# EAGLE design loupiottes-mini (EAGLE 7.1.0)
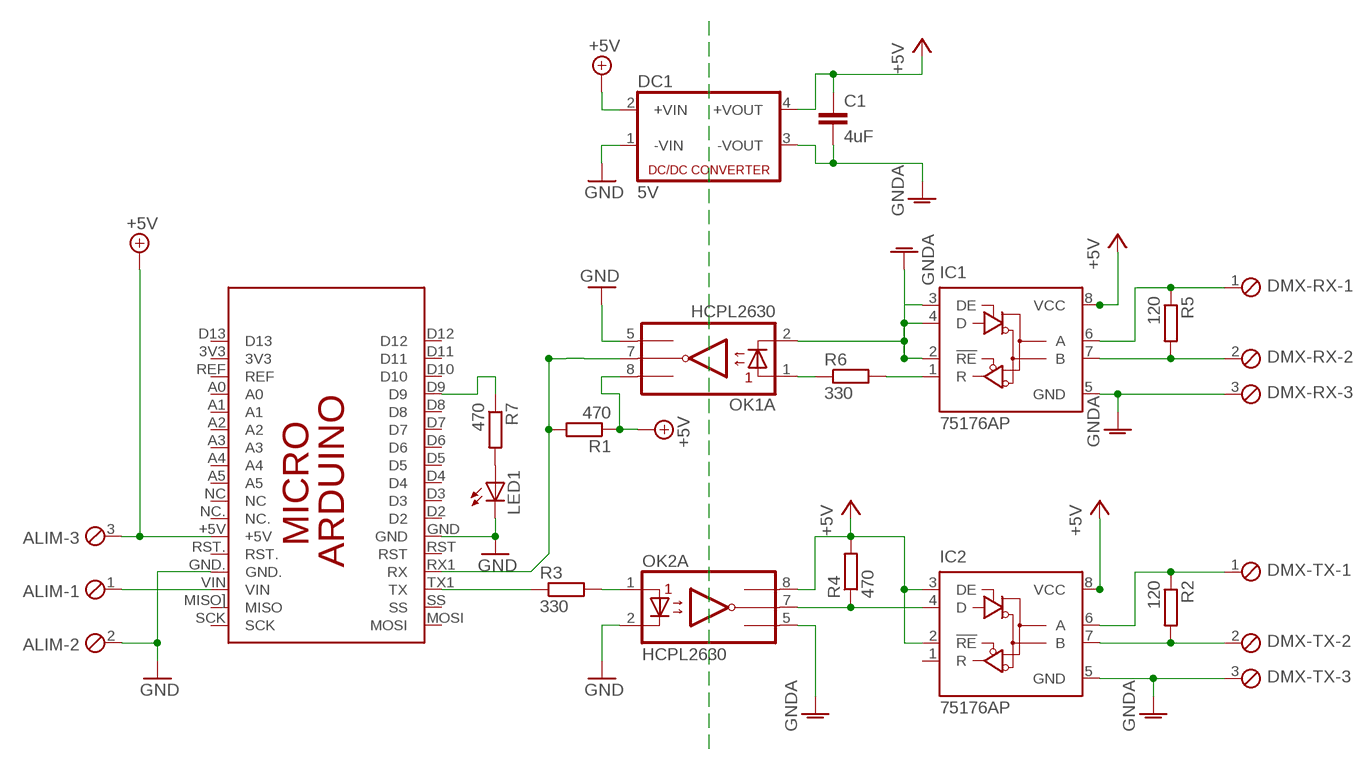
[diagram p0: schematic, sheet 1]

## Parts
ALIM  MPT3  [3POL254]
C1  4uF  C-EU025-024X044  [C025-024X044]
DC1  5V  NME  [NME]
DMX-RX  MPT3  [3POL254]
DMX-TX  MPT3  [3POL254]
IC1  75176AP  [DIL08]
IC2  75176AP  [DIL08]
LED1  LED3MM  [LED3MM]
OK1  HCPL2630  [DIL08]
OK2  HCPL2630  [DIL08]
PCB1  ARDUINO_MICRO  [ARDUINO_MICRO]
R1  470  R-EU_0207/10  [0207/10]
R2  120  R-EU_0207/10  [0207/10]
R3  330  R-EU_0207/10  [0207/10]
R4  470  R-EU_0207/10  [0207/10]
R5  120  R-EU_0207/10  [0207/10]
R6  330  R-EU_0207/10  [0207/10]
R7  470  R-EU_0207/10  [0207/10]

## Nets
+5V: ALIM.3 DC1.2(+VIN) OK1.8(A:VCC) PCB1.+5V R1.1
+5V-ISO: C1.1 DC1.4(+VOUT) IC1.8(VCC) IC2.2(!RE) IC2.3(DE) IC2.8(VCC) OK2.8(A:VCC) R4.2 ; supply symbol labelled +5V
GND: ALIM.2 DC1.1(-VIN) LED1.K(C) OK1.5(A:GND) OK2.2(A:C1) PCB1.GND PCB1.GND.
GND-ISO: C1.2 DC1.3(-VOUT) DMX-RX.3 DMX-TX.3 IC1.2(!RE) IC1.3(DE) IC1.4(D) IC1.5(GND) IC2.5(GND) OK1.2(A:C1) OK2.5(A:GND) ; supply symbol labelled GNDA
N$1: PCB1.TX1(TX) R3.1
N$2: OK2.1(A:A1) R3.2
N$3: OK1.7(A:VO1) PCB1.RX1(RX) R1.2
N$4: IC2.4(D) OK2.7(A:VO1) R4.1
N$5: DMX-TX.1 IC2.6(A) R2.1
N$6: DMX-TX.2 IC2.7(B) R2.2
N$7: DMX-RX.1 IC1.6(A) R5.1
N$8: DMX-RX.2 IC1.7(B) R5.2
N$9: OK1.1(A:A1) R6.1
N$10: IC1.1(R) R6.2
N$11: LED1.A R7.2
N$13: ALIM.1 PCB1.VIN
N$14: PCB1.D9 R7.1
Unconnected: IC2.1(R) OK1.3(B:C2) OK1.4(B:A2) OK1.6(B:VO2) OK2.3(B:C2) OK2.4(B:A2) OK2.6(B:VO2) PCB1.3V3 PCB1.A0 PCB1.A1 PCB1.A2 PCB1.A3 PCB1.A4 PCB1.A5 PCB1.D2 PCB1.D3 PCB1.D4 PCB1.D5 PCB1.D6 PCB1.D7 PCB1.D8 PCB1.D10 PCB1.D11 PCB1.D12 PCB1.D13 PCB1.MISO](MISO) PCB1.MOSI PCB1.NC PCB1.NC. PCB1.REF PCB1.RST PCB1.RST. PCB1.SCK PCB1.SS

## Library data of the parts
ALIM DMX-RX DMX-TX = con-phoenix-254:MPT3: PHOENIX CONNECTOR; OC_FARNELL: unknown; OC_NEWARK: unknown
C1 = rcl:C-EU: CAPACITOR, European symbol
DC1 = dc-dc-converter:NME: DC-DC CONVERTER; MF: C & D TECHNOLOGIES, INC; MPN: NME1205D; OC_FARNELL: 1021466; OC_NEWARK: 98B8198
IC1 IC2 = 751xx:75176A: DIFFERENTIAL BUS TRANSCEIVER Source: http://focus.ti.com/lit/ds/symlink/sn75176a.pdf
LED1 = led:LED: LED
OK1 OK2 = optocoupler:HCPL2630: HEWLETT PACKARD OPTO COUPLER; MF: AGILENT TECHNOLOGIES; MPN: HCPL-2630-000E; OC_FARNELL: 9994904; OC_NEWARK: 88H7813
PCB1 = E14_Arduino:ARDUINO_MICRO: Device for representing an Arduino Micro board with a footprint in an EAGLE design. Created by Dave Young for Element14. More EAGLE documentation at: http://www.element14.com/community/community/knode/cadsoft_eagle
R1-R7 = rcl:R-EU_: RESISTOR, European symbol

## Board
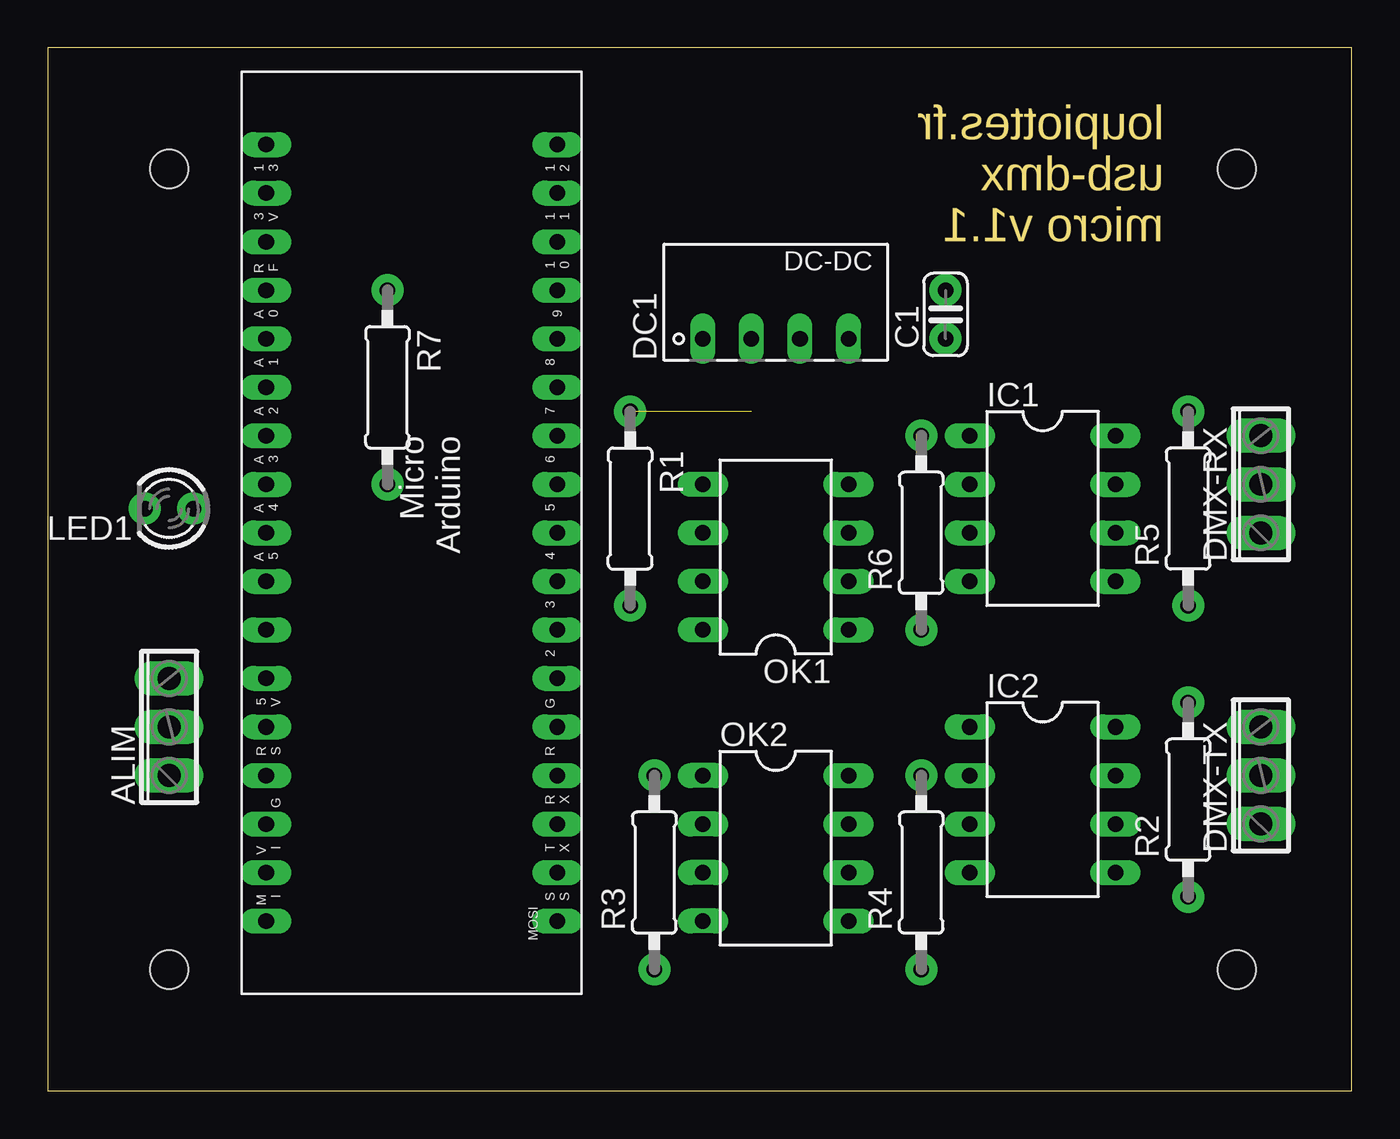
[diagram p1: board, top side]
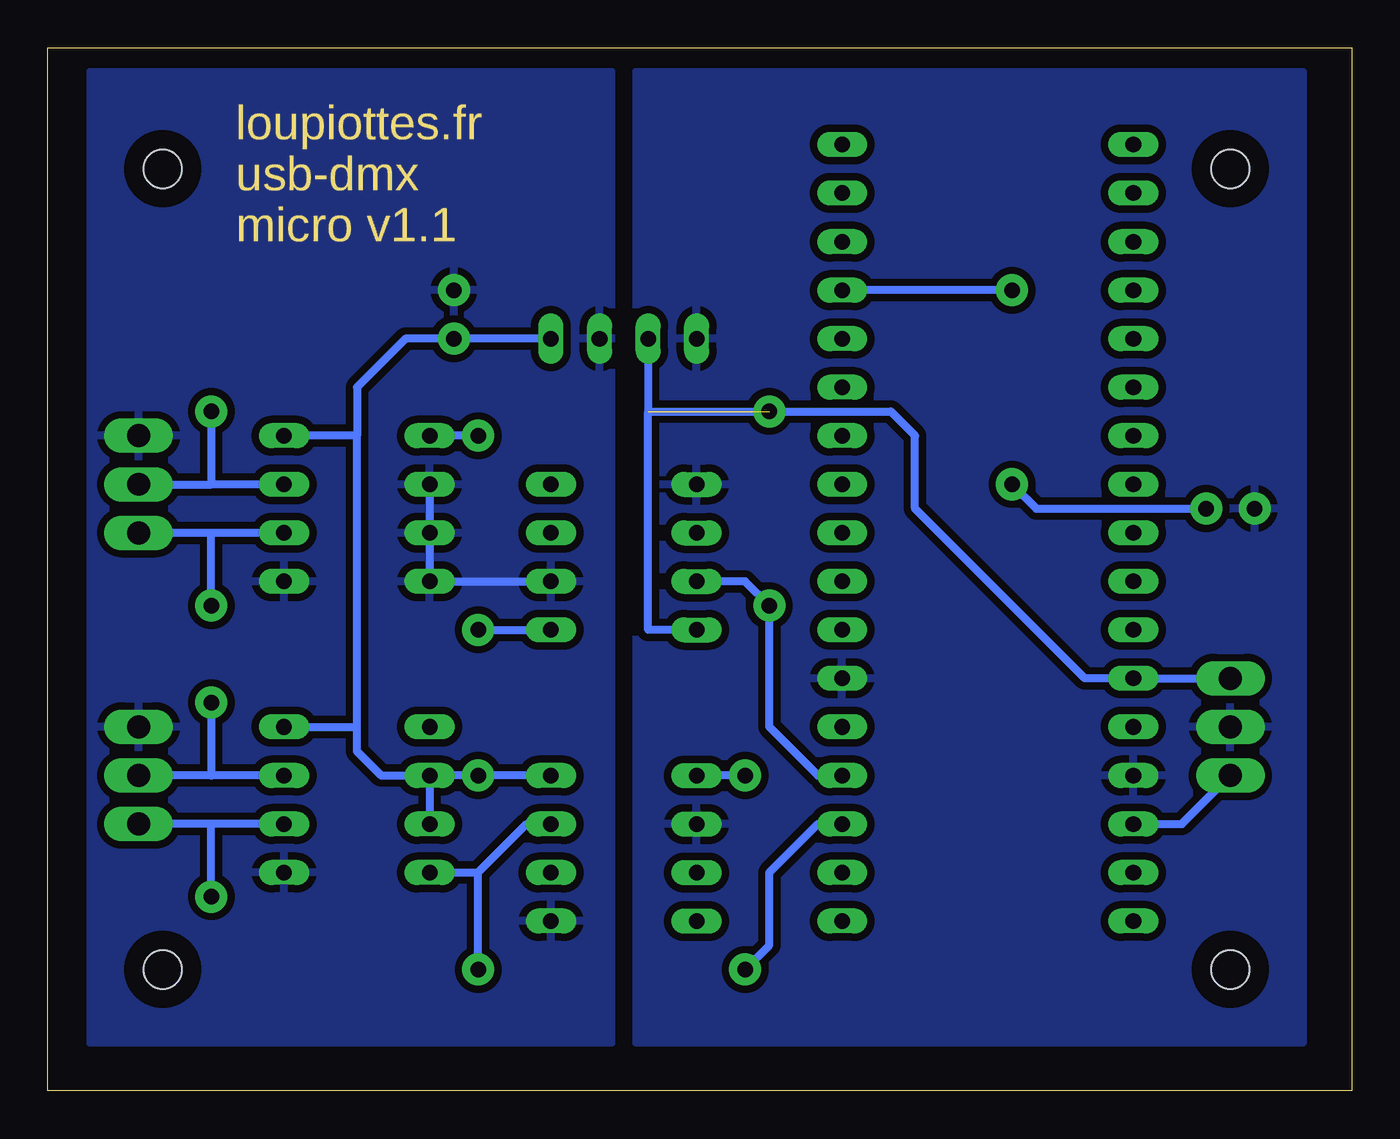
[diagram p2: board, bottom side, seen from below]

Size 68.25 x 54.6 mm. Coordinates in mm from the lower left corner, seen from the top.
Outline: 0,0 68.25,0 68.25,54.6 0,54.6 0,0
Copper layers (1*16): Top 0.035mm / dielectric 1.5mm / Bottom 0.035mm
Design rules "Gcode *": minimum track width 15mil, minimum drill 24mil, track to track 15mil, track to pad 15mil, pad to pad 15mil, via to via 15mil, smd to smd 8mil, copper to edge 40mil, drill to drill 8mil, minimum pad ring 10mil, minimum via ring 8mil, stop-mask expansion 4mil, vias tented up to drill 0mil, thermal gap 15mil
Holes 2 mm at 6.35,6.35 62.23,6.35 6.35,48.26 62.23,48.26

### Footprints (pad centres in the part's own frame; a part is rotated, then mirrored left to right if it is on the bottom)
3POL254 = drill 1.2 long: 1 -2.54,0; 2 0,0; 3 2.54,0
C025-024X044 = drill 0.813 pad 1.676: 1 -1.27,0; 2 1.27,0
NME = drill 0.813 long: 1 0,3.81; 2 0,1.27; 3 0,-1.27; 4 0,-3.81
DIL08 = drill 0.813 long: 1 -3.81,-3.81; 2 -1.27,-3.81; 3 1.27,-3.81; 4 3.81,-3.81; 5 3.81,3.81; 6 1.27,3.81; 7 -1.27,3.81; 8 -3.81,3.81
LED3MM = drill 0.813 pad 1.676: A -1.27,0; K 1.27,0
ARDUINO_MICRO = drill 0.813 long: 3V3 6.35,1.27; +5V 31.75,1.27; A0 11.43,1.27; A1 13.97,1.27; A2 16.51,1.27; A3 19.05,1.27; A4 21.59,1.27; A5 24.13,1.27; D2 29.21,16.51; D3 26.67,16.51; D4 24.13,16.51; D5 21.59,16.51; D6 19.05,16.51; D7 16.51,16.51; D8 13.97,16.51; D9 11.43,16.51; D10 8.89,16.51; D11 6.35,16.51; D12 3.81,16.51; D13 3.81,1.27; GND 31.75,16.51; GND. 36.83,1.27; MISO] 41.91,1.27; MOSI 44.45,16.51; NC 26.67,1.27; NC. 29.21,1.27; REF 8.89,1.27; RST 34.29,16.51; RST. 34.29,1.27; RX1 36.83,16.51; SCK 44.45,1.27; SS 41.91,16.51; TX1 39.37,16.51; VIN 39.37,1.27
0207/10 = drill 0.813 pad 1.676: 1 -5.08,0; 2 5.08,0

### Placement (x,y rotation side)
ALIM  6.35,19.05 90 top
C1  46.99,40.64 90 top
DC1  38.1,39.37 90 top
DMX-RX  63.5,31.75 90 top
DMX-TX  63.5,16.51 90 top
IC1  52.07,30.48 270 top
IC2  52.07,15.24 270 top
LED1  6.35,30.48 180 top
OK1  38.1,27.94 90 top
OK2  38.1,12.7 270 top
PCB1  10.16,53.34 270 top
R1  30.48,30.48 270 top
R2  59.69,15.24 90 top
R3  31.75,11.43 90 top
R4  45.72,11.43 90 top
R5  59.69,30.48 90 top
R6  45.72,29.21 90 top
R7  17.78,36.83 270 top

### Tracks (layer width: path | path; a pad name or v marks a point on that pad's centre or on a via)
+5V  (1 unrouted)
  Bottom 0.406: ALIM.3 PCB1.+5V 13.97,21.59 22.86,30.48 22.86,34.29 24.13,35.56 36.83,35.56 | DC1.2 36.83,35.56 | OK1.8 36.83,24.13 36.83,35.56
+5V-ISO
  Bottom 0.406: 52.07,34.29 IC1.8 | 52.07,19.05 52.07,17.78 50.8,16.51 IC2.2 | 52.07,19.05 52.07,34.29 | IC2.2 IC2.3 | IC2.2 R4.2 OK2.8 | DC1.4 C1.1 49.53,39.37 52.07,36.83 52.07,34.29 | IC2.8 52.07,19.05
GND
  pour Bottom (isolate 0.279): 37.47,2.54 2.54,2.54 2.54,53.34 37.47,53.34
GND-ISO
  Bottom 0.406: IC1.2 IC1.3 IC1.4 OK1.2
  pour Bottom (isolate 0.279): 38.73,2.54 38.73,53.34 66.04,53.34 66.04,2.54
N$1
  Bottom 0.406: PCB1.TX1 27.94,13.97 30.48,11.43 30.48,7.62 R3.1
N$2
  Bottom 0.406: R3.2 OK2.1
N$3
  Bottom 0.406: PCB1.RX1 27.94,16.51 30.48,19.05 R1.2 31.75,26.67 OK1.7
N$4
  Bottom 0.406: OK2.7 43.18,13.97 45.72,11.43 | R4.1 45.72,11.43 | IC2.4 45.72,11.43
N$5
  Bottom 0.406: IC2.6 59.69,13.97 | 59.69,13.97 DMX-TX.1 | R2.1 59.69,13.97
N$6
  Bottom 0.406: IC2.7 59.69,16.51 | 59.69,16.51 DMX-TX.2 | R2.2 59.69,16.51
N$7
  Bottom 0.406: IC1.6 59.69,29.21 | 59.69,29.21 DMX-RX.1 | R5.1 59.69,29.21
N$8
  Bottom 0.406: IC1.7 59.69,31.75 | R5.2 59.69,31.75 | DMX-RX.2 59.69,31.75
N$9
  Bottom 0.406: R6.1 OK1.1
N$10
  Bottom 0.406: R6.2 IC1.1
N$11
  Bottom 0.406: R7.2 16.51,30.48 LED1.A
N$13
  Bottom 0.406: PCB1.VIN 8.89,13.97 ALIM.1
N$14
  Bottom 0.406: R7.1 PCB1.D9

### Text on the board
Milling: loupiottes.fr / usb-dmx / micro v1.1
